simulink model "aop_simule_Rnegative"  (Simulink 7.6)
settings: Solver=ode14x  StartTime=0.0  StopTime=0.04  RelTol=1e-3
InitFcn:
  | clc
StopFcn:
  | close all, clc
  | load simul_Rnegative.mat
  | plot(x(2,:),x(3,:))
  | title('Caractéristique u=f(i)')
  | xlabel('courant (A)')
  | ylabel('tension (V)')
  | grid
  | delete *.mat
libraries: fl_lib x9, nesl_utility x4, elec_lib x1

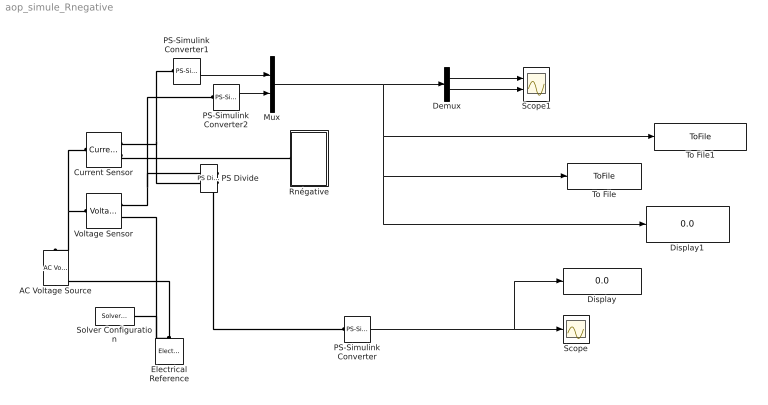
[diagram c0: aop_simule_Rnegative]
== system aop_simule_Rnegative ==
  AC Voltage Source : fl_lib/Electrical/Electrical Sources/AC Voltage Source  DialogController=NetworkEngine.DynNeDlgSource  SystemSampleTime=-1  amp=1 V  shift=0 rad  omega=60 Hz  i_Log=off  v_Log=off  LocalVarNames=|i|v  LocalVarDescs=|i|v  LocalVarLogging=[0 0]
  Current Sensor : fl_lib/Electrical/Electrical Sensors/Current Sensor  DialogController=NetworkEngine.DynNeDlgSource  SystemSampleTime=-1  i1_Log=off  v1_Log=off  LocalVarNames=|i1|v1  LocalVarDescs=|i1|v1  LocalVarLogging=[0 0]
  Demux : Demux  Outputs=2
  Display : Display
  Display1 : Display
  Electrical Reference : fl_lib/Electrical/Electrical Elements/Electrical Reference  DialogController=NetworkEngine.DynNeDlgSource  SystemSampleTime=-1  i_Log=off  LocalVarNames=|i  LocalVarDescs=|i  LocalVarLogging=0
  Mux : Mux  Inputs=2
  PS Divide : fl_lib/Physical Signals/Functions/PS Divide  DialogController=NetworkEngine.DynNeDlgSource  SystemSampleTime=-1  LocalVarLogging=[]
  PS-Simulink Converter : nesl_utility/PS-Simulink Converter  DialogController=NetworkEngine.DynNeUtilDlgSource  SystemSampleTime=-1  PhysicalDomain=network_engine_domain  LeftPortType=input  RightPortType=output  SubClassName=ps_output  Unit=1  AffineConversion=off
  PS-Simulink Converter1 : nesl_utility/PS-Simulink Converter  DialogController=NetworkEngine.DynNeUtilDlgSource  SystemSampleTime=-1  PhysicalDomain=network_engine_domain  LeftPortType=input  RightPortType=output  SubClassName=ps_output  Unit=1  AffineConversion=off
  PS-Simulink Converter2 : nesl_utility/PS-Simulink Converter  DialogController=NetworkEngine.DynNeUtilDlgSource  SystemSampleTime=-1  PhysicalDomain=network_engine_domain  LeftPortType=input  RightPortType=output  SubClassName=ps_output  Unit=1  AffineConversion=off
  Rnégative : Subsystem
  Scope : Scope
  Scope1 : Scope  NumInputPorts=2
  Solver Configuration : nesl_utility/Solver Configuration  DialogController=NetworkEngine.DynNeUtilDlgSource  SystemSampleTime=-1  PhysicalDomain=network_engine_domain  LeftPortType=input  RightPortType=generic  SubClassName=solver  Accelerate=off  Profile=off  ResidualTolerance=1e-9  MaxNonlinIter=3  MaxModeIter=2  DoFixedCost=off  UseLocalSampling=off  DoDC=off  LinearAlgebra=Sparse  LocalSolverSampleTime=.001  LocalSolverChoice=NE_BACKWARD_EULER_ADVANCER  UseLocalSolver=off
  To File : ToFile  Filename=Ve_Ie  MatrixName=x
  To File1 : ToFile  Filename=simul_Rnegative  MatrixName=x
  Voltage Sensor : fl_lib/Electrical/Electrical Sensors/Voltage Sensor  DialogController=NetworkEngine.DynNeDlgSource  SystemSampleTime=-1  i1_Log=off  v1_Log=off  LocalVarNames=|i1|v1  LocalVarDescs=|i1|v1  LocalVarLogging=[0 0]
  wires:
  PS-Simulink Converter/1 -> Scope/1, Display/1
  PS-Simulink Converter1/1 -> Mux/1
  PS-Simulink Converter2/1 -> Mux/2
  Mux/1 -> Demux/1, To File/1, Display1/1, To File1/1
  Demux/1 -> Scope1/1
  Demux/2 -> Scope1/2
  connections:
  Electrical Reference/LConn1 -- AC Voltage Source/RConn1 -- Voltage Sensor/RConn2 -- Solver Configuration/RConn1
  Current Sensor/LConn1 -- AC Voltage Source/LConn1 -- Voltage Sensor/LConn1
  PS-Simulink Converter1/LConn1 -- Current Sensor/RConn1 -- PS Divide/LConn2
  Voltage Sensor/RConn1 -- PS-Simulink Converter2/LConn1 -- PS Divide/LConn1
  PS Divide/RConn1 -- PS-Simulink Converter/LConn1
  Current Sensor/RConn2 -- Rnégative/LConn1

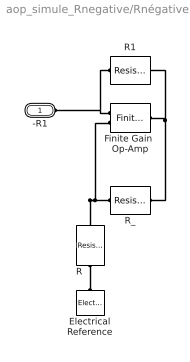
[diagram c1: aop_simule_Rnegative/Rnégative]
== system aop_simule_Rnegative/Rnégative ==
  Electrical Reference : fl_lib/Electrical/Electrical Elements/Electrical Reference  DialogController=NetworkEngine.DynNeDlgSource  SystemSampleTime=-1  i_Log=off  LocalVarNames=|i  LocalVarDescs=|i  LocalVarLogging=0
  Finite Gain  Op-Amp : elec_lib/Integrated Circuits/Finite Gain Op-Amp  DialogController=NetworkEngine.DynNeDlgSource  SystemSampleTime=-1  A=1000  Rin=1e+6 Ohm  Rout=100 Ohm  Vmin=-15 V  Vmax=15 V  LocalVarLogging=[]
  R : fl_lib/Electrical/Electrical Elements/Resistor  DialogController=NetworkEngine.DynNeDlgSource  SystemSampleTime=-1  R=1 kOhm  i_Log=off  v_Log=off  LocalVarNames=|i|v  LocalVarDescs=|i|v  LocalVarLogging=[0 0]
  R1 : fl_lib/Electrical/Electrical Elements/Resistor  DialogController=NetworkEngine.DynNeDlgSource  SystemSampleTime=-1  R=1 kOhm  i_Log=off  v_Log=off  LocalVarNames=|i|v  LocalVarDescs=|i|v  LocalVarLogging=[0 0]
  R_ : fl_lib/Electrical/Electrical Elements/Resistor  DialogController=NetworkEngine.DynNeDlgSource  SystemSampleTime=-1  R=1 kOhm  i_Log=off  v_Log=off  LocalVarNames=|i|v  LocalVarDescs=|i|v  LocalVarLogging=[0 0]
  -R1 : PMIOPort  Port=1  Side=Left
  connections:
  R_/RConn1 -- Finite Gain  Op-Amp/RConn1 -- R1/RConn1
  R_/LConn1 -- Finite Gain  Op-Amp/LConn2 -- R/LConn1
  R1/LConn1 -- -R1/RConn1 -- Finite Gain  Op-Amp/LConn1
  R/RConn1 -- Electrical Reference/LConn1
